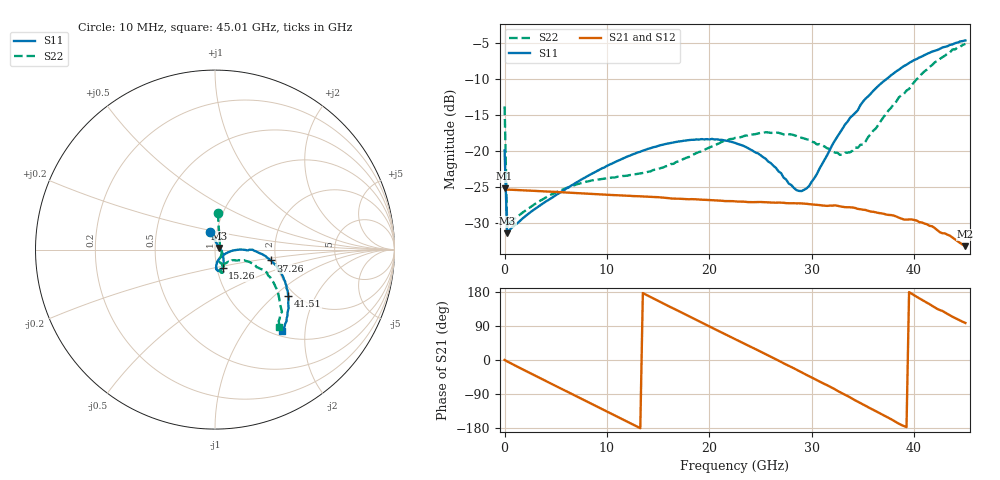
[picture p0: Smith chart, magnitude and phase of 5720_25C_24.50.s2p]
! Device:  ADRF5720
! Description: 0.5dB LSB GaAs MMIC 6-bit Digital Attenuator
! Frequency:  0.000009 -  40 GHz
! Ports:
!	RF1	= Port 1
!	RF2	= Port 2
! Vdd:  3.3 Volt
! Vss:  -3.3 Volt
! Control:  0/3.3 Volt
! State:  24.50 dB attenuation
! Data:  The device was measured using G-S-G Probes on a matrix board.
!  Data was collected using an calibrated 4 port network analyzer.
!  The reference plane for this measurement is at the launchers.
! Note:  Analog Devices supplies this data as a sample of measured data
!  for this product.  Your particular data for this product may vary.
!  Data was taken at 25 degrees C.
!  Analog Devices reserves the right to change this data at anytime.
# GHZ S DB R 45.0
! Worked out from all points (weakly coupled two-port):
!   181 points, 10 MHz to 45.01 GHz, reference 45 ohm
!   highest |S21| = -25.17 dB at 10 MHz (marker M1); lowest = -33.2 dB at 45.01 GHz (marker M2)
!   lowest |S11| = -31.5 dB at 260 MHz (marker M3), VSWR 1.05, Z = 47.3 + j0.871 ohm
!   |S11| at or under -10 dB: start of sweep to 37.29 GHz
!   |S22| runs from -30.6 to -5.1 dB; largest |S21 - S12| = 0.00011
!   S11 on the Smith chart (normalised r, x): 10 MHz: 0.93, +0.18; 15.26 GHz: 1.07, -0.22; 37.26 GHz: 1.87, -0.25; 41.51 GHz: 1.84, -1.24; 45.01 GHz: 1.09, -1.52
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0.01  -19.93 106.4  -25.17 0.1  -25.17 0.1  -13.80 85.6
0.26  -31.47 20.1  -25.37 -3.8  -25.37 -3.8  -30.62 15.6
1.26  -30.06 1.7  -25.43 -17.7  -25.44 -17.7  -29.12 -8.0
3.51  -27.54 -19.4  -25.59 -48.3  -25.59 -48.3  -26.90 -38.1
7.76  -23.77 -44.0  -25.91 -105.6  -25.91 -105.6  -24.35 -68.4
12.01  -20.76 -58.6  -26.23 -162.9  -26.23 -162.9  -23.44 -74.5
15.26  -19.18 -67.2  -26.46 152.6  -26.46 152.6  -22.38 -68.9
20.26  -18.31 -79.7  -26.86 85.1  -26.86 85.1  -19.36 -63.6
22.76  -19.01 -85.3  -27.04 51.8  -27.03 51.8  -18.18 -66.3
25.51  -21.09 -84.9  -27.13 15.1  -27.14 15.1  -17.39 -71.8
28.51  -25.44 -58.1  -27.29 -25.5  -27.29 -25.4  -17.91 -76.2
29.51  -25.20 -34.9  -27.35 -39.5  -27.35 -39.5  -18.37 -74.9
30.26  -23.78 -18.5  -27.46 -49.7  -27.45 -49.7  -18.80 -74.4
32.76  -17.47 0.1  -27.71 -84.8  -27.70 -84.8  -20.53 -60.0
33.76  -15.35 -0.7  -27.84 -98.8  -27.84 -98.8  -20.17 -46.3
35.01  -13.13 -1.8  -28.17 -117.0  -28.17 -116.9  -19.11 -33.3
37.26  -10.03 -11.0  -28.84 -149.3  -28.84 -149.3  -14.85 -20.1
37.76  -9.44 -13.3  -28.92 -156.3  -28.91 -156.2  -13.98 -19.7
40.26  -7.19 -25.9  -29.69 166.6  -29.70 166.6  -10.00 -23.8
41.51  -6.32 -32.3  -30.42 147.4  -30.39 147.4  -8.29 -30.5
43.76  -5.15 -43.8  -32.06 114.0  -32.07 114.0  -5.85 -43.0
45.01  -4.61 -50.7  -33.25 97.7  -33.25 97.7  -5.08 -50.3
